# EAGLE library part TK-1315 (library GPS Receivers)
TK-1315 GPS receiver Producted by San Jose Technology,Inc.
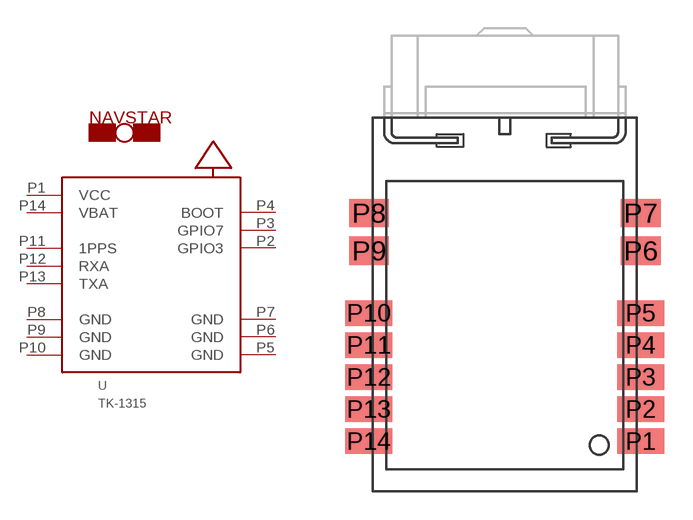
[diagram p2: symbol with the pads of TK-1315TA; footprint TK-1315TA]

Designator prefix U

## TK-1315-TA  [TK-1315TA]
P1  VCC
P2  GPIO3
P3  GPIO7
P4  BOOT  nc
P5  GND
P6  GND
P7  GND
P8  GND
P9  GND
P10  GND
P11  1PPS
P12  RXA
P13  TXA
P14  VBAT

## Footprint TK-1315TA (pad centres in mm)
smd 2.5 x 1.35: P1 7.2,-6.8; P2 7.2,-5.1; P3 7.2,-3.4; P4 7.2,-1.7; P5 7.2,0; P10 -7.2,0; P11 -7.2,-1.7; P12 -7.2,-3.4; P13 -7.2,-5.1; P14 -7.2,-6.8
smd 2.1 x 1.5: P6 7.2,3.3; P7 7.2,5.3; P8 -7.2,5.3; P9 -7.2,3.3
